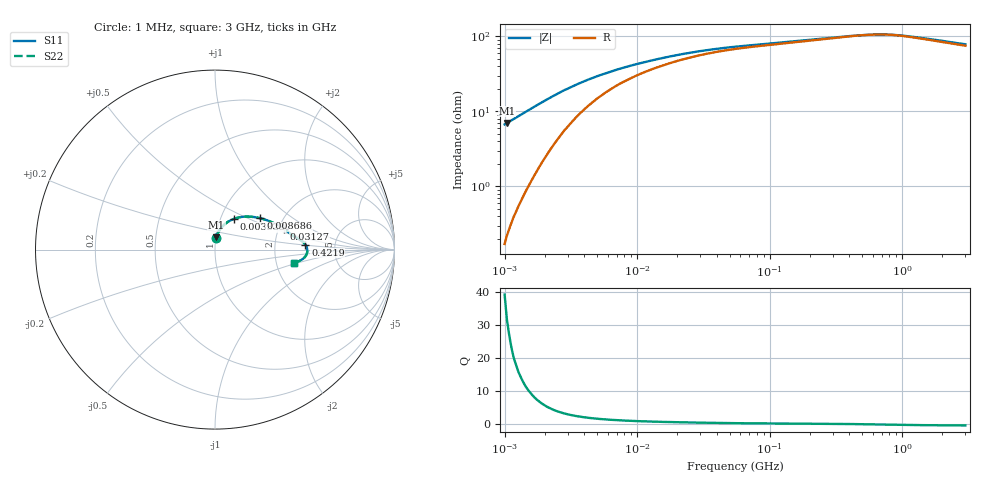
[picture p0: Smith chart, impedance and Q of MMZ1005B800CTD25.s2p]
! S-Parameter Data Generated by TDK Corporation
! Copyright(C) 2025 TDK Corporation.
! All Rights Reserved.
! TDK P/N: MMZ1005B800CTD25 (Chip Bead)
! Property: |Z|=80ohm at 100MHz
! Size(LxWxT): 1x0.5x0.5mm
! Model Type: s2p (Touchstone File Format Version 1.0)
! Frequency: DC=Yes Start=1MHz Stop=3000MHz 202points Log-sweep
! Model Generated on Feb. 6, 2025
! Terms and conditions regarding TDK Simulation Models:
! 1)This simulation model is being provided solely for informational
!  purposes. Please refer to the specifications of the products in
!  terms of detailed characteristics of such products.
! 2)In no event shall TDK Corporation of any of its subsidiaries be
!  liable for any loss or damage arising, directly or indirectly,
!  from any information contained in this simulation model, including,
!  but not limited to loss or damages arising from any inaccuracies,
!  omissions or errors in connection with such information.
! 3)Any and all copyrights on this simulation model are owned by
!  TDK Corporation.  Duplication or redistribution of this simulation
!  model without prior written permission from TDK Corporation
!  is prohibited.
! 4)This simulation model is subject to any modification or change
!  without any prior notice.
! 5)Neither TDK Corporation nor any of its subsidiaries shall make any
!  warranty, express or implied, including but not limited to the
!  correctness, implied warranties of merchantability and fitness for
!  a particular purpose with respect to this simulation models.
! 6)The use of this simulation model shall be deemed to have consented
!  to the terms and conditions hereof.
! Port Assignments:
!  1 ---@@@--- 2
! Applicable Conditions:
!  Temperature = 25 degC
!  DC Bias Current = 0 A
!  Small Signal Operation
# Hz S MA R 50
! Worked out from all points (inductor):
!   201 points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, 1 MHz to 3 GHz, reference 50 ohm
!   read as one part in series: L = 1.08 uH near 1.041 MHz
!   highest Q = 31.6 at 1.041 MHz (marker M1), where L = 1.07 uH
!   self-resonance near 643.7 MHz
!   S11 on the Smith chart (normalised r, x): 1 MHz: 1.00, +0.13; 3.323 MHz: 1.15, +0.41; 8.686 MHz: 1.54, +0.59; 31.27 MHz: 2.14, +0.59; 421.9 MHz: 3.02, +0.22; 3 GHz: 2.50, -0.47
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1000000  0.0667 84.7  0.9961 -3.8  0.9961 -3.8  0.0667 84.7
1040844  0.06959 84.2  0.9954 -4.0  0.9954 -4.0  0.06959 84.2
1492300  0.1006 78.8  0.9855 -5.7  0.9855 -5.7  0.1006 78.8
2055611  0.1371 71.9  0.9663 -7.8  0.9663 -7.8  0.1371 71.9
2831560  0.1794 63.1  0.9328 -9.9  0.9328 -9.9  0.1794 63.1
3323290  0.1998 58.6  0.9121 -10.8  0.9121 -10.8  0.1998 58.6
3900413  0.2203 54.0  0.8887 -11.6  0.8887 -11.6  0.2203 54.0
4959344  0.2496 47.5  0.8513 -12.5  0.8513 -12.5  0.2496 47.5
5592179  0.2629 44.4  0.8328 -12.8  0.8328 -12.8  0.2629 44.4
6831390  0.2843 39.6  0.8017 -13.1  0.8017 -13.1  0.2843 39.6
8686058  0.3074 34.6  0.7669 -13.1  0.7669 -13.1  0.3074 34.6
1.461624e7  0.3516 25.8  0.7003 -12.6  0.7003 -12.6  0.3516 25.8
2.013356e7  0.3752 21.5  0.6653 -11.9  0.6653 -11.9  0.3752 21.5
3.127247e7  0.4021 16.7  0.6256 -10.6  0.6256 -10.6  0.4021 16.7
5.477226e7  0.4277 12.1  0.5888 -8.8  0.5888 -8.8  0.4277 12.1
2.136344e8  0.4788 6.4  0.527 -5.8  0.527 -5.8  0.4788 6.4
4.219165e8  0.5046 3.1  0.4969 -3.2  0.4969 -3.2  0.5046 3.1
6.049187e8  0.5134 0.5  0.4867 -0.6  0.4867 -0.6  0.5134 0.5
8.005644e8  0.5133 -1.9  0.4873 2.0  0.4873 2.0  0.5133 -1.9
9.779672e8  0.5081 -3.7  0.494 3.8  0.494 3.8  0.5081 -3.7
1.402151e9  0.4903 -6.2  0.5154 5.9  0.5154 5.9  0.4903 -6.2
3e9  0.4445 -9.7  0.5667 7.6  0.5667 7.6  0.4445 -9.7
